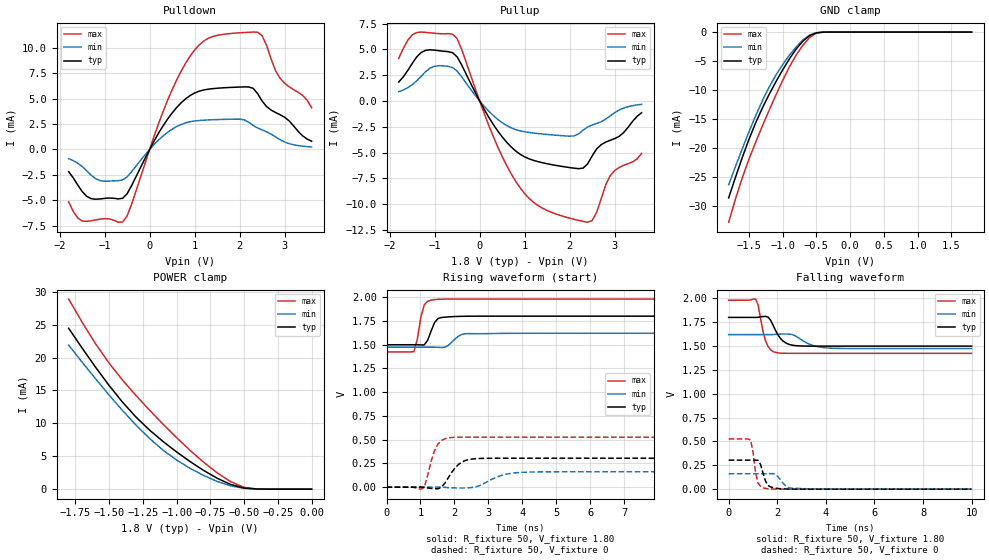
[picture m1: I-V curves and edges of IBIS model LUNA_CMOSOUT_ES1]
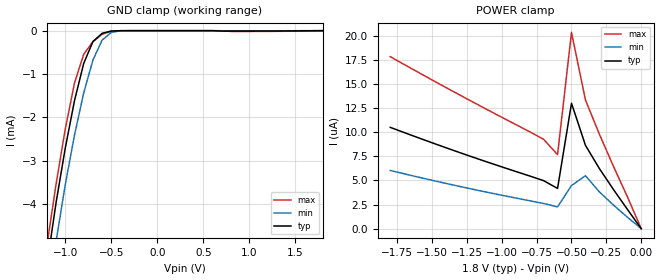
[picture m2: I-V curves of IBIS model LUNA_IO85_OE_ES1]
[IBIS Ver]   3.2
[Comment Char]   |_char
[File name]   sg-9101cx_18v_c.ibs
[File Rev]   1.0
[Date]   2020/01/21 2:13:43
[Source]
[Notes]
[Disclaimer]
This information is for modeling purposes only, and is not guaranteed.
Property of SEIKO EPSON Corp.,
unauthorized reproduction and/or distribution is strictly prohibited.
[Copyright]
Copyright 2020, SEIKO EPSON Corp.
[Component]   SG-9101CA
Si_location Pin
Timing_location Pin
[Manufacturer]   SEIKO EPSON Corp.
| 7050 PKG
| 7050 PKG
[Package]
R_pkg   224m   NA   NA
L_pkg   5.5n   NA   NA
C_pkg   0.144p   NA   NA
[Pin] signal_name   model_name
1   OE   LUNA_IO85_OE_ES1
2   VSS   GND
3   OUT   LUNA_CMOSOUT_ES1
4   VDD   POWER
[Component]   SG-9101CB
Si_location Pin
Timing_location Pin
[Manufacturer]   SEIKO EPSON Corp.
| 5032 PKG
| 5032 PKG
[Package]
R_pkg   200m   NA   NA
L_pkg   2.16n   NA   NA
C_pkg   1.23p   NA   NA
[Pin] signal_name   model_name
1   OE   LUNA_IO85_OE_ES1
2   VSS   GND
3   OUT   LUNA_CMOSOUT_ES1
4   VDD   POWER
[Component]   SG-9101CE
Si_location Pin
Timing_location Pin
[Manufacturer]   SEIKO EPSON Corp.
| 3225 PKG
| 3225 PKG
[Package]
R_pkg   177m   NA   NA
L_pkg   4.5n   NA   NA
C_pkg   0.64p   NA   NA
[Pin] signal_name   model_name
1   OE   LUNA_IO85_OE_ES1
2   VSS   GND
3   OUT   LUNA_CMOSOUT_ES1
4   VDD   POWER
[Component]   SG-9101CG
Si_location Pin
Timing_location Pin
[Manufacturer]   SEIKO EPSON Corp.
| 2520 PKG
| 2520 PKG
[Package]
R_pkg   238m   NA   NA
L_pkg   2.1n   NA   NA
C_pkg   0.38p   NA   NA
[Pin] signal_name   model_name
1   OE   LUNA_IO85_OE_ES1
2   VSS   GND
3   OUT   LUNA_CMOSOUT_ES1
4   VDD   POWER
| Models and submodels in the file (2): LUNA_CMOSOUT_ES1 (3-state), LUNA_IO85_OE_ES1 (Input)
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[Model]   LUNA_CMOSOUT_ES1
Model_type 3-state
Enable Active-High
Polarity Non-Inverting
Vmeas=0.90
C_comp   2.5p   2.0p   3.0p
[Temperature Range] 25   105   -40
[Voltage Range]   1.80   1.62   1.98
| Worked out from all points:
|   slope of the pulldown table from 0 to 0.27 V, typ, clamps not added: 128 ohm
|   slope of the pullup table from 0 to 0.27 V, typ, clamps not added: 132 ohm
|   GND clamp passes 1 mA (typ) near -0.64 V on its own axis
|   POWER clamp passes 1 mA (typ) near -0.63 V on its own axis
|   falling waveform, R_fixture 50, V_fixture 1.80: 20-80 % time 427ps typ, 663ps min, 296ps max; typ from 1.8 V to 1.5 V
|   falling waveform, R_fixture 50, V_fixture 0: 20-80 % time 241ps typ, 334ps min, 196ps max; typ from 0.304 V to 0 V
|   rising waveform, R_fixture 50, V_fixture 1.80: 20-80 % time 208ps typ, 276ps min, 183ps max; typ from 1.5 V to 1.8 V
|   rising waveform, R_fixture 50, V_fixture 0: 20-80 % time 387ps typ, 613ps min, 271ps max; typ from 0 V to 0.304 V
[Pullup]
-1.8V     1.832mA    895.6uA    4.119mA
-1.5V     3.632mA    1.567mA    6.401mA
-1.2V     4.909mA    2.841mA    6.65mA
-500mV    4.267mA    2.895mA    6.036mA
200mV     -1.556mA   -979.5uA   -2.339mA
600mV     -3.999mA   -2.382mA   -6.252mA
1.1V      -5.611mA   -3.053mA   -9.449mA
1.6V      -6.173mA   -3.286mA   -10.8mA
2.3V      -6.51mA    -2.828mA   -11.68mA
2.5V      -5.338mA   -2.332mA   -11.59mA
2.9V      -3.818mA   -1.459mA   -7.254mA
3.6V      -1.139mA   -334.4uA   -5.088mA
[Pulldown]
-1.8V     -2.186mA   -910.2uA   -5.151mA
-1.6V     -3.49mA    -1.348mA   -6.738mA
-1.3V     -4.847mA   -2.531mA   -7.02mA
-600mV    -4.81mA    -3.001mA   -7.141mA
600mV     4.119mA    2.245mA    6.829mA
1V        5.55mA     2.797mA    9.777mA
1.4V      5.979mA    2.918mA    11.1mA
2.1V      6.15mA     2.914mA    11.5mA
2.4V      5.492mA    2.103mA    11.53mA
2.5V      4.761mA    1.916mA    11.18mA
2.9V      3.413mA    945.5uA    6.997mA
3.6V      802.6uA    241.5uA    4.102mA
[GND Clamp]
-1.8V     -28.67mA   -26.41mA   -32.88mA
-1.6V     -21.75mA   -20.22mA   -25.25mA
-1.5V     -18.58mA   -17.27mA   -22mA
-1.4V     -15.69mA   -14.46mA   -19.04mA
-1.2V     -10.77mA   -9.503mA   -13.52mA
-1.1V     -8.591mA   -7.44mA    -10.88mA
-900mV    -4.635mA   -4.001mA   -6.009mA
-700mV    -1.565mA   -1.365mA   -2.263mA
-600mV    -601.2uA   -521.6uA   -925.2uA
-500mV    -121.4uA   -116.4uA   -188.8uA
-400mV    -10.57uA   -14.63uA   -13.06uA
1.8V      99.8pA     105.8nA    71.35pA
[POWER Clamp]
-1.8V     24.46mA    21.89mA    28.9mA
-1.6V     18.52mA    16.76mA    22.08mA
-1.5V     15.75mA    14.3mA     19.15mA
-1.3V     10.93mA    9.714mA    14.21mA
-1.1V     7.236mA    5.92mA     9.861mA
-1V       5.655mA    4.424mA    7.824mA
-900mV    4.191mA    3.162mA    5.894mA
-700mV    1.665mA    1.179mA    2.483mA
-600mV    721.7uA    498.7uA    1.143mA
-500mV    167.2uA    126.9uA    275.1uA
-400mV    16.41uA    18.75uA    19.76uA
0V        99.8pA     596.4pA    86.97pA
[Falling Waveform]
R_fixture=50
V_fixture=1.80
V_fixture_min=1.62
V_fixture_max=1.98
0s        1.8V       1.62V      1.98V
1.111ns   1.8V       1.62V      1.991V
1.212ns   1.801V     1.62V      1.931V
1.515ns   1.81V      1.62V      1.556V
1.717ns   1.774V     1.62V      1.463V
1.919ns   1.668V     1.622V     1.434V
2.323ns   1.537V     1.626V     1.424V
2.828ns   1.503V     1.594V     1.423V
4.141ns   1.499V     1.479V     1.423V
10ns      1.499V     1.474V     1.423V
[Falling Waveform]
R_fixture=50
V_fixture=0
V_fixture_min=0
V_fixture_max=0
0s        304.2mV    161.5mV    526mV
909.1ps   304.2mV    161.5mV    513.8mV
1.01ns    304.1mV    161.5mV    373.6mV
1.111ns   304.4mV    161.5mV    168.7mV
1.212ns   302.1mV    161.5mV    63.15mV
1.515ns   86.43mV    161.3mV    7.846mV
1.919ns   11.11mV    155.4mV    819.9uV
2.323ns   2.484mV    40.24mV    76.55uV
2.626ns   847.4uV    9.649mV    15.03uV
10ns      0V         0V         0V
[Rising Waveform]
R_fixture=50
V_fixture=1.80
V_fixture_min=1.62
V_fixture_max=1.98
0s        1.499V     1.474V     1.423V
808.1ps   1.499V     1.474V     1.427V
909.1ps   1.499V     1.474V     1.56V
1.01ns    1.497V     1.474V     1.786V
1.111ns   1.497V     1.474V     1.919V
1.313ns   1.643V     1.474V     1.969V
1.515ns   1.775V     1.472V     1.977V
1.919ns   1.794V     1.525V     1.98V
2.323ns   1.799V     1.615V     1.98V
10ns      1.8V       1.62V      1.98V
[Rising Waveform]
R_fixture=50
V_fixture=0
V_fixture_min=0
V_fixture_max=0
0s        0V         0V         0V
1.111ns   -1.623mV   3.37uV     -3.622mV
1.414ns   -16.1mV    87.23uV    382.7mV
1.616ns   -1.527mV   272.6uV    490.9mV
1.818ns   97.27mV    -5.304mV   518.7mV
2.222ns   263.9mV    -9.753mV   525.7mV
2.626ns   299.3mV    2.417mV    526mV
3.333ns   304.1mV    116.8mV    526mV
3.939ns   304.2mV    154.6mV    526mV
10ns      304.2mV    161.5mV    526mV
[Ramp]
R_load=50
dV/dt_r   1.825E-1/3.855E-10   9.690E-2/6.118E-10   3.156E-1/2.649E-10
dV/dt_f   1.806E-1/4.219E-10   8.789E-2/6.603E-10   3.339E-1/2.936E-10
|[End   LUNA_CMOSOUT_ES1
[Model]   LUNA_IO85_OE_ES1
Model_type Input
Enable Active-Low
Polarity Non-Inverting
Vinh=1.39
Vinl=0.48
C_comp   2.5p   2.0p   3.0p
[Model Spec]
[Temperature Range] 25   105   -40
[Voltage Range]   1.80   1.62   1.98
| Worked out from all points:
|   GND clamp passes 1 mA (typ) near -0.83 V on its own axis
[GND Clamp]
-1.8V     -17.06mA   -17.31mA   -17.53mA
-1.2V     -5.408mA   -6.351mA   -4.953mA
-1.1V     -3.959mA   -4.854mA   -3.533mA
-1V       -2.702mA   -3.543mA   -2.264mA
-900mV    -1.611mA   -2.406mA   -1.207mA
-800mV    -755.6uA   -1.435mA   -543.8uA
-700mV    -251.6uA   -679.9uA   -253.8uA
-600mV    -60.29uA   -218.4uA   -84.58uA
-500mV    -8.175uA   -39.66uA   -10.45uA
-400mV    -667.8nA   -4.047uA   -594nA
800mV     -9.61uA    -4.857uA   -17.73uA
1.8V      72.89pA    2.202uA    -5.276uA
[POWER Clamp]
-1.8V     10.5uA     6.032uA    17.83uA
-1.3V     7.877uA    4.371uA    13.84uA
-700mV    4.977uA    2.609uA    9.265uA
-600mV    4.168uA    2.258uA    7.669uA
-500mV    13uA       4.465uA    20.34uA
-400mV    8.645uA    5.49uA     13.35uA
-300mV    6.229uA    3.813uA    9.792uA
-200mV    4.08uA     2.459uA    6.49uA
-100mV    2.02uA     1.199uA    3.335uA
0V        72.85pA    181.7pA    73.98pA
